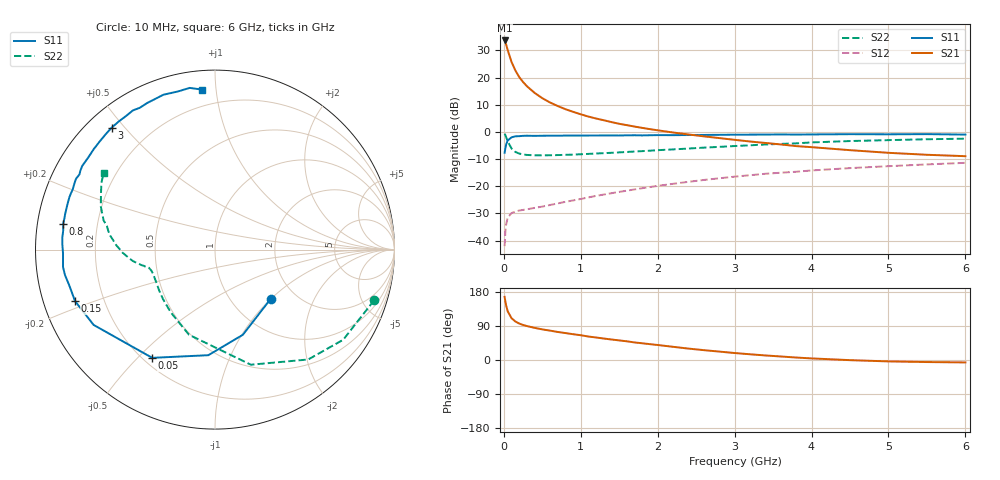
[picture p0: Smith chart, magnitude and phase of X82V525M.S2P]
! SIEMENS Small Signal Semiconductors
! BFP136W
! Si NPN RF Bipolar Junction Transistor in SOT343
! VCE = 2.5 V  IC = 25 mA
! Common Emitter S-Parameters:  September  1994
# GHz  S  MA  R  50
!  f  S11  S21  S12  S22
! GHz  MAG  ANG  MAG  ANG  MAG  ANG  MAG  ANG
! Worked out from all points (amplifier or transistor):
!   40 points, 10 MHz to 6 GHz, reference 50 ohm
!   highest |S21| = 33.7 dB at 10 MHz (marker M1)
!   |S21| within 3 dB of that: start of sweep to 44.78 MHz
!   unconditionally stable (mu >= 1): 809.6 MHz to 2.787 GHz
!   at 200 MHz: K = 0.38, MSG = 24.6 dB, |S12| = -28.9 dB
!   at 1.5 GHz: K = 1.17, MAG = 10.1 dB, |S12| = -22.1 dB
!   at 6 GHz: K = 0.98, MSG = 1.2 dB, |S12| = -11.4 dB
!   S11 on the Smith chart (normalised r, x): 10 MHz: 1.50, -1.00; 50 MHz: 0.24, -0.55; 150 MHz: 0.10, -0.18; 800 MHz: 0.08, +0.08; 3 GHz: 0.07, +0.46; 6 GHz: 0.10, +0.92
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0.01  0.4142 -41.5  48.3 166.6  0.0079 76.1  0.9303 -17.7
0.02  0.4994 -71.9  44.53 154.2  0.0147 66.5  0.8733 -35.1
0.03  0.5895 -93.6  40.67 143.9  0.0198 56.9  0.8027 -49.7
0.05  0.6971 -120.1  32.16 128.7  0.0265 43.2  0.6717 -72.7
0.1  0.7961 -148.2  19.41 110.3  0.0321 30.0  0.496 -107.0
0.15  0.8309 -159.8  13.52 101.6  0.0342 27.1  0.4277 -125.2
0.2  0.8361 -166.2  10.24 96.2  0.0358 26.0  0.4002 -136.3
0.25  0.8479 -170.4  8.292 92.4  0.0367 26.5  0.3863 -143.5
0.3  0.8522 -173.5  6.951 89.6  0.0377 28.0  0.3774 -148.5
0.4  0.847 -178.5  5.236 84.8  0.04 30.9  0.3716 -154.8
0.5  0.8513 177.8  4.182 80.8  0.0423 34.1  0.3707 -158.7
0.6  0.8531 175.4  3.487 77.5  0.0452 37.3  0.3723 -161.0
0.7  0.8524 172.7  3.001 74.0  0.0483 40.0  0.3752 -162.5
0.8  0.8578 170.5  2.626 71.1  0.0517 42.4  0.379 -163.7
1.1  0.8593 163.9  1.917 61.9  0.0624 47.8  0.3946 -166.0
1.5  0.8608 157.0  1.413 51.7  0.0788 51.9  0.4207 -168.3
2.2  0.8729 144.3  0.977 34.8  0.111 52.5  0.4771 -173.8
3  0.8907 130.3  0.716 18.4  0.1504 48.4  0.5502 177.5
3.2  0.8928 126.9  0.667 15.1  0.1598 46.9  0.5677 175.0
4.5  0.9095 108.4  0.462 -0.4  0.216 35.4  0.6802 159.3
5.5  0.9119 98.9  0.38 -5.4  0.2526 27.2  0.7339 149.6
6  0.8943 94.6  0.358 -6.4  0.2702 22.6  0.7524 145.6
